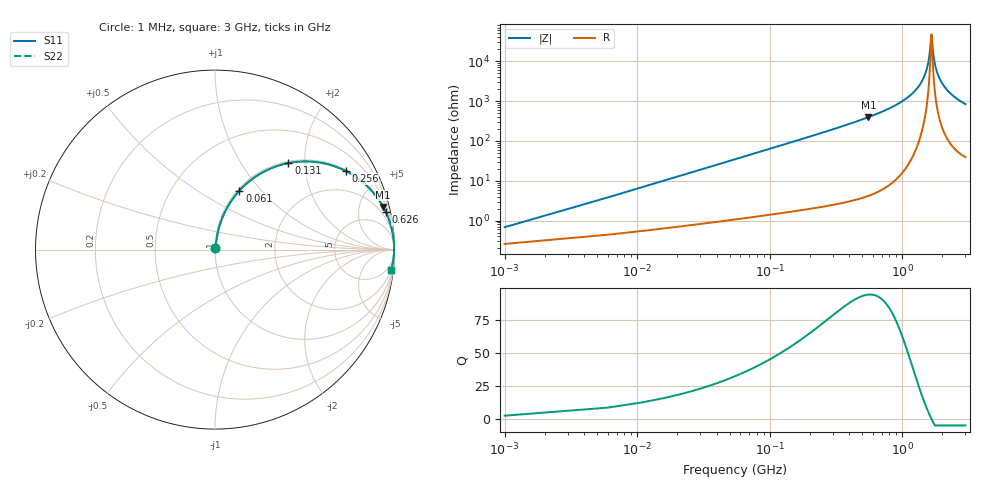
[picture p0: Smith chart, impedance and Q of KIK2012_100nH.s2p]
!version-2
!date-01.2022
!Series
# MHz S RI R 50
!Freq ReS11 ImS11 ReS21 ImS21 ReS12 ImS12 ReS22 ImS22
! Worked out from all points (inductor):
!   601 points, 1 MHz to 3 GHz, reference 50 ohm
!   read as one part in series: L = 100 nH near 16 MHz
!   highest Q = 94.6 at 556 MHz (marker M1), where L = 113 nH
!   self-resonance near 1.661 GHz
!   S11 on the Smith chart (normalised r, x): 1 MHz: 1.01, +0.01; 61 MHz: 1.02, +0.77; 131 MHz: 1.03, +1.66; 256 MHz: 1.04, +3.30; 626 MHz: 1.10, +9.16; 3 GHz: 2, -17
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1  0.00262 0.00625  0.9974 -0.00625  0.9974 -0.00625  0.00262 0.00625
21  0.0238 0.1279  0.9762 -0.1279  0.9762 -0.1279  0.0238 0.1279
26  0.0331 0.1568  0.9669 -0.1568  0.9669 -0.1568  0.0331 0.1568
41  0.0699 0.2375  0.9301 -0.2375  0.9301 -0.2375  0.0699 0.2375
61  0.1356 0.3281  0.8644 -0.3281  0.8644 -0.3281  0.1356 0.3281
131  0.4087 0.4821  0.5913 -0.4821  0.5913 -0.4821  0.4087 0.4821
256  0.7281 0.4382  0.2719 -0.4382  0.2719 -0.4382  0.7281 0.4382
501  0.9206 0.2651  0.0794 -0.2651  0.0794 -0.2651  0.9206 0.2651
556  0.9371 0.2376  0.0629 -0.2376  0.0629 -0.2376  0.9371 0.2376
626  0.9525 0.2074  0.0475 -0.2074  0.0475 -0.2074  0.9525 0.2074
1001  0.9883 0.1001  0.0117 -0.1001  0.0117 -0.1001  0.9883 0.1001
1311  0.9962 0.0457  0.00379 -0.0457  0.00379 -0.0457  0.9962 0.0457
1501  0.9977 0.0196  0.00227 -0.0196  0.00227 -0.0196  0.9977 0.0196
1586  0.9979 0.00908  0.00208 -0.00908  0.00208 -0.00908  0.9979 0.00908
1651  0.9979 0.00143  0.0021 -0.00143  0.0021 -0.00143  0.9979 0.00143
1666  0.9979 -0.000295  0.00212 0.000295  0.00212 0.000295  0.9979 -0.000295
1726  0.9977 -0.00703  0.00227 0.00703  0.00227 0.00703  0.9977 -0.00703
1781  0.9975 -0.013  0.00248 0.013  0.00248 0.013  0.9975 -0.013
1871  0.997 -0.0224  0.00298 0.0224  0.00298 0.0224  0.997 -0.0224
2001  0.996 -0.0353  0.00399 0.0353  0.00399 0.0353  0.996 -0.0353
2501  0.9897 -0.079  0.0103 0.079  0.0103 0.079  0.9897 -0.079
3000  0.9806 -0.1164  0.0194 0.1164  0.0194 0.1164  0.9806 -0.1164
